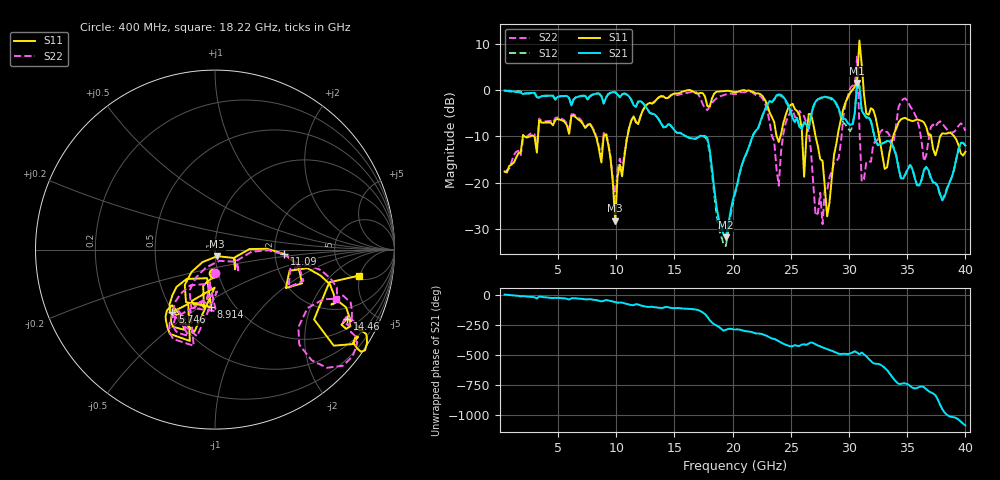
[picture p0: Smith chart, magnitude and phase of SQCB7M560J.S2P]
! Network Analyzer HP8722ES.07.66: Jul 25, 2000 Serial No. US39175408
! 27 Oct 2004  11:13:01
! Frequency  S11  S21  S12  S22
# HZ  S  DB R  50
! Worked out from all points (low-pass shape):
!   201 points, 400 MHz to 40 GHz, reference 50 ohm
!   highest |S21| = 1.56 dB at 30.69 GHz (marker M1); lowest = -31.8 dB at 19.41 GHz (marker M2)
!   |S21| within 3 dB of the highest: start of sweep to 3.182 GHz; 3.462 GHz to 4.625 GHz (1.163 GHz wide, 28.8 % of centre)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
!   lowest |S11| = -28.2 dB at 9.904 GHz (marker M3), VSWR 1.08, Z = 51.1 - j3.76 ohm
!   |S11| at or under -10 dB: start of sweep to 1.967 GHz; 9.156 GHz to 10.95 GHz (1.798 GHz wide, 17.9 % of centre); 27.13 GHz to 29.01 GHz (1.886 GHz wide, 6.72 % of centre)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
!   |S22| runs from -29.0 to 7.2 dB; largest |S21 - S12| = 0.33
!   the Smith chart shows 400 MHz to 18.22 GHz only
!   S11 on the Smith chart (normalised r, x): 400 MHz: 0.95, -0.25; 5.746 GHz: 0.50, -0.42; 8.914 GHz: 0.78, -0.56; 11.09 GHz: 2.25, -0.13; 14.46 GHz: 1.42, -3.55; 18.22 GHz: 5.60, -4.85
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4e8  -17.57 -93.9  -0.10 0.2  -0.04 1.1  -17.82 -90.0
5.746e9  -7.50 -124.3  -1.22 -34.8  -1.23 -35.0  -7.17 -120.2
7.132e9  -7.29 -128.3  -1.17 -37.2  -1.24 -37.8  -7.07 -122.6
8.914e9  -9.90 -94.0  -2.86 -52.2  -2.87 -51.9  -9.29 -89.1
9.904e9  -28.22 -71.2  -0.46 -62.6  -0.46 -63.1  -23.47 -68.9
1.1092e10  -8.28 -3.6  -1.34 -83.1  -1.28 -83.6  -8.17 -4.2
1.3666e10  -1.50 -26.9  -6.37 -110.7  -6.36 -110.4  -1.55 -24.1
1.4458e10  -1.60 -27.5  -7.36 -105.0  -7.24 -106.1  -1.69 -26.6
1.822e10  -1.76 -10.2  -16.82 126.0  -17.93 126.2  -2.77 -22.1
1.9408e10  -0.15 -19.6  -31.78 66.2  -33.71 65.7  -0.91 -24.9
2.02e10  -0.42 -22.1  -22.02 68.4  -22.60 68.7  -0.84 -28.9
2.5744e10  -5.37 -54.2  -7.91 -67.9  -7.96 -66.8  -4.46 -12.3
2.6932e10  -7.37 -16.1  -3.45 -44.2  -3.70 -46.1  -20.44 -139.1
2.812e10  -27.26 31.2  -1.55 -93.7  -1.52 -95.1  -21.65 97.2
2.9506e10  -4.03 99.8  -6.10 -132.9  -6.99 -136.4  -5.81 158.6
3.0496e10  0.73 46.1  -4.85 -112.1  -4.94 -105.6  0.93 116.5
3.0694e10  2.34 27.6  1.56 -124.0  1.57 -120.3  7.24 113.9
3.0892e10  10.76 -9.6  1.02 -136.9  0.79 -153.8  -8.03 134.3
3.109e10  5.52 -66.2  -4.40 -123.1  -4.53 -122.3  -19.75 -82.7
3.1288e10  -0.99 -77.9  -5.18 -138.1  -5.20 -136.6  -19.19 -24.2
3.3466e10  -13.61 -146.5  -11.03 65.2  -10.94 64.6  -9.66 99.9
4e10  -13.30 29.5  -11.95 -9.8  -12.02 -10.2  -8.76 118.7
